|Texas Instruments Incorporated
|ADC12DL3200 6.4-GSPS, Single-Channel or 3.2-GSPS, Dual-Channel
|12-bit Analog-to-Digital Converter (ADC) with LVDS Interface
[IBIS Ver]   4.1
[File name]   adc12dl3200.ibs
[Date]   06/13/2018
[File Rev]   1.1
[Source]
| Texas Instruments Incorporated.
| Analog-eLab Design Center, HPA
| 12500 TI Blvd
| Dallas, TX -75243
[Notes]   Revision History:
|| Rev 1.1: 06/13/2018
| - Included slow and fast corners for OUT_LVDS
| Rev 1.0: 05/15/2018
| - Initial version of the model
| - Model generated from simulations in SPECTRE
| - Warnings regarding combined Non-monotonicity of various models
|   have been reviewed and considered minor and can be ignored.
| - C_comp although listed in numerical order of value are
|   obtained from varying PVT conditions. For PVT conditions for
|   each specific value refer the buffer description under
|   respective [Model]. IBIS model user is responsible for using
|   appropriate C_comp to simulate for Signal Integrity.
[Disclaimer]
| This model is designed as an aid for customers of Texas Instruments.
| TI and its licensors and suppliers make no warranties, either expressed
| or implied, with respect to this  model, including the warranties of
| merchantability or fitness for a particular purpose. The model is
| provided solely on an "as is" basis. The entire risk as to its quality
| and performance is with the customer.
| This model is subject to change without notice. Texas Instruments
| Incorporated is not responsible for updating this model.
[Copyright]
(C) Copyright 2018 Texas Instruments Incorporated.All rights reserved.
|  Component ADC12DL3200ACF 256-pin FCBGA - ACF package
|  Part # ADC12DL3200ACF
[Component]   ADC12DL3200ACF
[Manufacturer]  TI
[Package]   |256 FCBGA- ACF package
|   typ   min   max
R_pkg   0.05   0.04   0.06
L_pkg   1.0nH   0.8nH   1.2nH
C_pkg   0.2pF   0.16pF   0.24pF
[Pin] signal_name  model_name   R_pin   L_pin   C_pin
A1   AGND   GND   NA   NA   NA
A2   AGND   GND   NA   NA   NA
A3   AGND   GND   NA   NA   NA
A4   INA+   NC   NA   NA   NA
A5   INA-   NC   NA   NA   NA
A6   AGND   GND   NA   NA   NA
A7   AGND   GND   NA   NA   NA
A8   ORA1   NC   NA   NA   NA
A9   DA0+   OUT_LVDS   NA   NA   NA
A10   DA0-   OUT_LVDS   NA   NA   NA
A11   DA6+   OUT_LVDS   NA   NA   NA
A12   DA6-   OUT_LVDS   NA   NA   NA
A13   DC0+   OUT_LVDS   NA   NA   NA
A14   DC0-   OUT_LVDS   NA   NA   NA
A15   DGND   GND   NA   NA   NA
A16   DGND   GND   NA   NA   NA
B1   CALSTAT   OUTPUT   NA   NA   NA
B2   CALTRIG   INPUT   NA   NA   NA
B3   AGND   GND   NA   NA   NA
B4   AGND   GND   NA   NA   NA
B5   AGND   GND   NA   NA   NA
B6   AGND   GND   NA   NA   NA
B7   AGND   GND   NA   NA   NA
B8   ORA0   NC   NA   NA   NA
B9   DA1+   OUT_LVDS   NA   NA   NA
B10   DA1-   OUT_LVDS   NA   NA   NA
B11   DA7+   OUT_LVDS   NA   NA   NA
B12   DA7-   OUT_LVDS   NA   NA   NA
B13   DC1+   OUT_LVDS   NA   NA   NA
B14   DC1-   OUT_LVDS   NA   NA   NA
B15   DC7+   OUT_LVDS   NA   NA   NA
B16   DC7-   OUT_LVDS   NA   NA   NA
C1   AGND   GND   NA   NA   NA
C2   AGND   GND   NA   NA   NA
C3   AGND   GND   NA   NA   NA
C4   AGND   GND   NA   NA   NA
C5   AGND   GND   NA   NA   NA
C6   AGND   GND   NA   NA   NA
C7   AGND   GND   NA   NA   NA
C8   ORB1   NC   NA   NA   NA
C9   DA2+   OUT_LVDS   NA   NA   NA
C10   DA2-   OUT_LVDS   NA   NA   NA
C11   DA8+   OUT_LVDS   NA   NA   NA
C12   DA8-   OUT_LVDS   NA   NA   NA
C13   DC2+   OUT_LVDS   NA   NA   NA
C14   DC2-   OUT_LVDS   NA   NA   NA
C15   DC8+   OUT_LVDS   NA   NA   NA
C16   DC8-   OUT_LVDS   NA   NA   NA
D1   TMSTP+   SYNCB   NA   NA   NA
D2   BG   NC   NA   NA   NA
D3   AGND   GND   NA   NA   NA
D4   AGND   GND   NA   NA   NA
D5   AGND   GND   NA   NA   NA
D6   AGND   GND   NA   NA   NA
D7   DGND   GND   NA   NA   NA
D8   ORB0   NC   NA   NA   NA
D9   DA3+   OUT_LVDS   NA   NA   NA
D10   DA3-   OUT_LVDS   NA   NA   NA
D11   DA9+   OUT_LVDS   NA   NA   NA
D12   DA9-   OUT_LVDS   NA   NA   NA
D13   DC3+   OUT_LVDS   NA   NA   NA
D14   DC3-   OUT_LVDS   NA   NA   NA
D15   DC9+   OUT_LVDS   NA   NA   NA
D16   DC9-   OUT_LVDS   NA   NA   NA
E1   TMSTP-   SYNCB   NA   NA   NA
E2   SYNCSEb   INPUT   NA   NA   NA
E3   AGND   GND   NA   NA   NA
E4   VA11   POWER   NA   NA   NA
E5   VA11   POWER   NA   NA   NA
E6   VA11   POWER   NA   NA   NA
E7   DGND   GND   NA   NA   NA
E8   VD11   POWER   NA   NA   NA
E9   DA4+   OUT_LVDS   NA   NA   NA
E10   DA4-   OUT_LVDS   NA   NA   NA
E11   DA10+   OUT_LVDS   NA   NA   NA
E12   DA10-   OUT_LVDS   NA   NA   NA
E13   DC4+   OUT_LVDS   NA   NA   NA
E14   DC4-   OUT_LVDS   NA   NA   NA
E15   DC10+   OUT_LVDS   NA   NA   NA
E16   DC10-   OUT_LVDS   NA   NA   NA
F1   AGND   GND   NA   NA   NA
F2   AGND   GND   NA   NA   NA
F3   VA11   POWER   NA   NA   NA
F4   VA11   POWER   NA   NA   NA
F5   VA11   POWER   NA   NA   NA
F6   VA11   POWER   NA   NA   NA
F7   DGND   GND   NA   NA   NA
F8   VD11   POWER   NA   NA   NA
F9   DA5+   OUT_LVDS   NA   NA   NA
F10   DA5-   OUT_LVDS   NA   NA   NA
F11   DA11+   OUT_LVDS   NA   NA   NA
F12   DA11-   OUT_LVDS   NA   NA   NA
F13   DC5+   OUT_LVDS   NA   NA   NA
F14   DC5-   OUT_LVDS   NA   NA   NA
F15   DC11+   OUT_LVDS   NA   NA   NA
F16   DC11-   OUT_LVDS   NA   NA   NA
G1   AGND   GND   NA   NA   NA
G2   AGND   GND   NA   NA   NA
G3   VA19   POWER   NA   NA   NA
G4   VA19   POWER   NA   NA   NA
G5   VA19   POWER   NA   NA   NA
G6   VA19   POWER   NA   NA   NA
G7   DGND   GND   NA   NA   NA
G8   VD11   POWER   NA   NA   NA
G9   DACLK+   OUT_LVDS   NA   NA   NA
G10   DACLK-   OUT_LVDS   NA   NA   NA
G11   VLVDS   POWER   NA   NA   NA
G12   VLVDS   POWER   NA   NA   NA
G13   DC6+   OUT_LVDS   NA   NA   NA
G14   DC6-   OUT_LVDS   NA   NA   NA
G15   DCCLK+   OUT_LVDS   NA   NA   NA
G16   DCCLK-   OUT_LVDS   NA   NA   NA
H1   CLK+   DEVCLK   NA   NA   NA
H2   AGND   GND   NA   NA   NA
H3   VA19   POWER   NA   NA   NA
H4   VA19   POWER   NA   NA   NA
H5   VA19   POWER   NA   NA   NA
H6   VA19   POWER   NA   NA   NA
H7   DGND   GND   NA   NA   NA
H8   DGND   GND   NA   NA   NA
H9   DASTR+   OUT_LVDS   NA   NA   NA
H10   DASTR-   OUT_LVDS   NA   NA   NA
H11   VLVDS   POWER   NA   NA   NA
H12   VLVDS   POWER   NA   NA   NA
H13   VLVDS   POWER   NA   NA   NA
H14   DGND   GND   NA   NA   NA
H15   DCSTR+   OUT_LVDS   NA   NA   NA
H16   DCSTR-   OUT_LVDS   NA   NA   NA
J1   CLK-   DEVCLK   NA   NA   NA
J2   AGND   GND   NA   NA   NA
J3   VA19   POWER   NA   NA   NA
J4   VA19   POWER   NA   NA   NA
J5   VA19   POWER   NA   NA   NA
J6   VA19   POWER   NA   NA   NA
J7   DGND   GND   NA   NA   NA
J8   DGND   GND   NA   NA   NA
J9   DBSTR+   OUT_LVDS   NA   NA   NA
J10   DBSTR-   OUT_LVDS   NA   NA   NA
J11   VLVDS   POWER   NA   NA   NA
J12   VLVDS   POWER   NA   NA   NA
J13   VLVDS   POWER   NA   NA   NA
J14   DGND   GND   NA   NA   NA
J15   DDSTR+   OUT_LVDS   NA   NA   NA
J16   DDSTR-   OUT_LVDS   NA   NA   NA
K1   AGND   GND   NA   NA   NA
K2   AGND   GND   NA   NA   NA
K3   VA19   POWER   NA   NA   NA
K4   VA19   POWER   NA   NA   NA
K5   VA19   POWER   NA   NA   NA
K6   VA19   POWER   NA   NA   NA
K7   DGND   GND   NA   NA   NA
K8   VD11   POWER   NA   NA   NA
K9   DBCLK+   OUT_LVDS   NA   NA   NA
K10   DBCLK-   OUT_LVDS   NA   NA   NA
K11   VLVDS   POWER   NA   NA   NA
K12   VLVDS   POWER   NA   NA   NA
K13   DD6+   OUT_LVDS   NA   NA   NA
K14   DD6-   OUT_LVDS   NA   NA   NA
K15   DDCLK+   OUT_LVDS   NA   NA   NA
K16   DDCLK-   OUT_LVDS   NA   NA   NA
L1   AGND   GND   NA   NA   NA
L2   AGND   GND   NA   NA   NA
L3   VA11   POWER   NA   NA   NA
L4   VA11   POWER   NA   NA   NA
L5   VA11   POWER   NA   NA   NA
L6   VA11   POWER   NA   NA   NA
L7   DGND   GND   NA   NA   NA
L8   VD11   POWER   NA   NA   NA
L9   DB5+   OUT_LVDS   NA   NA   NA
L10   DB5-   OUT_LVDS   NA   NA   NA
L11   DB11+   OUT_LVDS   NA   NA   NA
L12   DB11-   OUT_LVDS   NA   NA   NA
L13   DD5+   OUT_LVDS   NA   NA   NA
L14   DD5-   OUT_LVDS   NA   NA   NA
L15   DD11+   OUT_LVDS   NA   NA   NA
L16   DD11-   OUT_LVDS   NA   NA   NA
M1   SYSREF+   SYSREF   NA   NA   NA
M2   TDIODE+   NC   NA   NA   NA
M3   AGND   GND   NA   NA   NA
M4   VA11   POWER   NA   NA   NA
M5   VA11   POWER   NA   NA   NA
M6   VA11   POWER   NA   NA   NA
M7   DGND   GND   NA   NA   NA
M8   VD11   POWER   NA   NA   NA
M9   DB4+   OUT_LVDS   NA   NA   NA
M10   DB4-   OUT_LVDS   NA   NA   NA
M11   DB10+   OUT_LVDS   NA   NA   NA
M12   DB10-   OUT_LVDS   NA   NA   NA
M13   DD4+   OUT_LVDS   NA   NA   NA
M14   DD4-   OUT_LVDS   NA   NA   NA
M15   DD10+   OUT_LVDS   NA   NA   NA
M16   DD10-   OUT_LVDS   NA   NA   NA
N1   SYSREF-   SYSREF   NA   NA   NA
N2   TDIODE-   NC   NA   NA   NA
N3   AGND   GND   NA   NA   NA
N4   AGND   GND   NA   NA   NA
N5   AGND   GND   NA   NA   NA
N6   AGND   GND   NA   NA   NA
N7   DGND   GND   NA   NA   NA
N8   SDO   OUTPUT   NA   NA   NA
N9   DB3+   OUT_LVDS   NA   NA   NA
N10   DB3-   OUT_LVDS   NA   NA   NA
N11   DB9+   OUT_LVDS   NA   NA   NA
N12   DB9-   OUT_LVDS   NA   NA   NA
N13   DD3+   OUT_LVDS   NA   NA   NA
N14   DD3-   OUT_LVDS   NA   NA   NA
N15   DD9+   OUT_LVDS   NA   NA   NA
N16   DD9-   OUT_LVDS   NA   NA   NA
P1   AGND   GND   NA   NA   NA
P2   AGND   GND   NA   NA   NA
P3   AGND   GND   NA   NA   NA
P4   AGND   GND   NA   NA   NA
P5   AGND   GND   NA   NA   NA
P6   AGND   GND   NA   NA   NA
P7   AGND   GND   NA   NA   NA
P8   SDI   INPUT   NA   NA   NA
P9   DB2+   OUT_LVDS   NA   NA   NA
P10   DB2-   OUT_LVDS   NA   NA   NA
P11   DB8+   OUT_LVDS   NA   NA   NA
P12   DB8-   OUT_LVDS   NA   NA   NA
P13   DD2+   OUT_LVDS   NA   NA   NA
P14   DD2-   OUT_LVDS   NA   NA   NA
P15   DD8+   OUT_LVDS   NA   NA   NA
P16   DD8-   OUT_LVDS   NA   NA   NA
R1   PD   INPUT   NA   NA   NA
R2   AGND   GND   NA   NA   NA
R3   AGND   GND   NA   NA   NA
R4   AGND   GND   NA   NA   NA
R5   AGND   GND   NA   NA   NA
R6   AGND   GND   NA   NA   NA
R7   AGND   GND   NA   NA   NA
R8   SCSb   INPUT   NA   NA   NA
R9   DB1+   OUT_LVDS   NA   NA   NA
R10   DB1-   OUT_LVDS   NA   NA   NA
R11   DB7+   OUT_LVDS   NA   NA   NA
R12   DB7-   OUT_LVDS   NA   NA   NA
R13   DD1+   OUT_LVDS   NA   NA   NA
R14   DD1-   OUT_LVDS   NA   NA   NA
R15   DD7+   OUT_LVDS   NA   NA   NA
R16   DD7-   OUT_LVDS   NA   NA   NA
T1   AGND   GND   NA   NA   NA
T2   AGND   GND   NA   NA   NA
T3   AGND   GND   NA   NA   NA
T4   INB+   NC   NA   NA   NA
T5   INB-   NC   NA   NA   NA
T6   AGND   GND   NA   NA   NA
T7   AGND   GND   NA   NA   NA
T8   SCLK   INPUT   NA   NA   NA
T9   DB0+   OUT_LVDS   NA   NA   NA
T10   DB0-   OUT_LVDS   NA   NA   NA
T11   DB6+   OUT_LVDS   NA   NA   NA
T12   DB6-   OUT_LVDS   NA   NA   NA
T13   DD0+   OUT_LVDS   NA   NA   NA
T14   DD0-   OUT_LVDS   NA   NA   NA
T15   DGND   GND   NA   NA   NA
T16   DGND   GND   NA   NA   NA
[Diff pin]  inv_pin  vdiff  tdelay_typ  tdelay_min  tdelay_max
A9   A10   0.0s   0.0s   0.0s   0.0s
A11   A12   0.0s   0.0s   0.0s   0.0s
A13   A14   0.0s   0.0s   0.0s   0.0s
B9   B10   0.0s   0.0s   0.0s   0.0s
B11   B12   0.0s   0.0s   0.0s   0.0s
B13   B14   0.0s   0.0s   0.0s   0.0s
B15   B16   0.0s   0.0s   0.0s   0.0s
C9   C10   0.0s   0.0s   0.0s   0.0s
C11   C12   0.0s   0.0s   0.0s   0.0s
C13   C14   0.0s   0.0s   0.0s   0.0s
C15   C16   0.0s   0.0s   0.0s   0.0s
D9   D10   0.0s   0.0s   0.0s   0.0s
D11   D12   0.0s   0.0s   0.0s   0.0s
D13   D14   0.0s   0.0s   0.0s   0.0s
D15   D16   0.0s   0.0s   0.0s   0.0s
E9   E10   0.0s   0.0s   0.0s   0.0s
E11   E12   0.0s   0.0s   0.0s   0.0s
E13   E14   0.0s   0.0s   0.0s   0.0s
E15   E16   0.0s   0.0s   0.0s   0.0s
F9   F10   0.0s   0.0s   0.0s   0.0s
F11   F12   0.0s   0.0s   0.0s   0.0s
F13   F14   0.0s   0.0s   0.0s   0.0s
F15   F16   0.0s   0.0s   0.0s   0.0s
G9   G10   0.0s   0.0s   0.0s   0.0s
G13   G14   0.0s   0.0s   0.0s   0.0s
G15   G16   0.0s   0.0s   0.0s   0.0s
H9   H10   0.0s   0.0s   0.0s   0.0s
H15   H16   0.0s   0.0s   0.0s   0.0s
J9   J10   0.0s   0.0s   0.0s   0.0s
J15   J16   0.0s   0.0s   0.0s   0.0s
K9   K10   0.0s   0.0s   0.0s   0.0s
K13   K14   0.0s   0.0s   0.0s   0.0s
K15   K16   0.0s   0.0s   0.0s   0.0s
L9   L10   0.0s   0.0s   0.0s   0.0s
L11   L12   0.0s   0.0s   0.0s   0.0s
L13   L14   0.0s   0.0s   0.0s   0.0s
L15   L16   0.0s   0.0s   0.0s   0.0s
M9   M10   0.0s   0.0s   0.0s   0.0s
M11   M12   0.0s   0.0s   0.0s   0.0s
M13   M14   0.0s   0.0s   0.0s   0.0s
M15   M16   0.0s   0.0s   0.0s   0.0s
N9   N10   0.0s   0.0s   0.0s   0.0s
N11   N12   0.0s   0.0s   0.0s   0.0s
N13   N14   0.0s   0.0s   0.0s   0.0s
N15   N16   0.0s   0.0s   0.0s   0.0s
P9   P10   0.0s   0.0s   0.0s   0.0s
P11   P12   0.0s   0.0s   0.0s   0.0s
P13   P14   0.0s   0.0s   0.0s   0.0s
P15   P16   0.0s   0.0s   0.0s   0.0s
R9   R10   0.0s   0.0s   0.0s   0.0s
R11   R12   0.0s   0.0s   0.0s   0.0s
R13   R14   0.0s   0.0s   0.0s   0.0s
R15   R16   0.0s   0.0s   0.0s   0.0s
T9   T10   0.0s   0.0s   0.0s   0.0s
T11   T12   0.0s   0.0s   0.0s   0.0s
T13   T14   0.0s   0.0s   0.0s   0.0s
D1   E1   0.0s   0.0s   0.0s   0.0s
H1   J1   0.0s   0.0s   0.0s   0.0s
M1   N1   0.0s   0.0s   0.0s   0.0s
[Model Selector] OUT_LVDS
OUT_LVDS_1P9_HIGH 1.9V Input configured for High swing mode
OUT_LVDS_1P9_LOW  1.9V Input configured for Low swing mode
OUT_LVDS_1P1_HIGH 1.1V Input configured for High swing mode
OUT_LVDS_1P1_LOW  1.1V Input configured for Low swing mode
[Model Selector] SYNCB
SYNCB_JESD   Input configured for JESD204B LVDS levels
SYNCB_PECL   Input configured for LVCMOS levels
[Model Selector] DEVCLK
DEVCLK_JESD   Input configured for JESD204B LVDS levels
DEVCLK_PECL   Input configured for LVCMOS levels
[Model Selector] SYSREF
SYSREF_JESD   Input configured for JESD204B LVDS levels
SYSREF_PECL   Input configured for LVCMOS levels
| Models and submodels in the file (12): OUT_LVDS_1P9_HIGH (Output), OUT_LVDS_1P9_LOW (Output), OUT_LVDS_1P1_HIGH (Output), OUT_LVDS_1P1_LOW (Output), SYNCB_JESD (Input), SYNCB_PECL (Input), DEVCLK_JESD (Input), DEVCLK_PECL (Input), SYSREF_JESD (Input), SYSREF_PECL (Input), INPUT (Input), OUTPUT (3-state)
